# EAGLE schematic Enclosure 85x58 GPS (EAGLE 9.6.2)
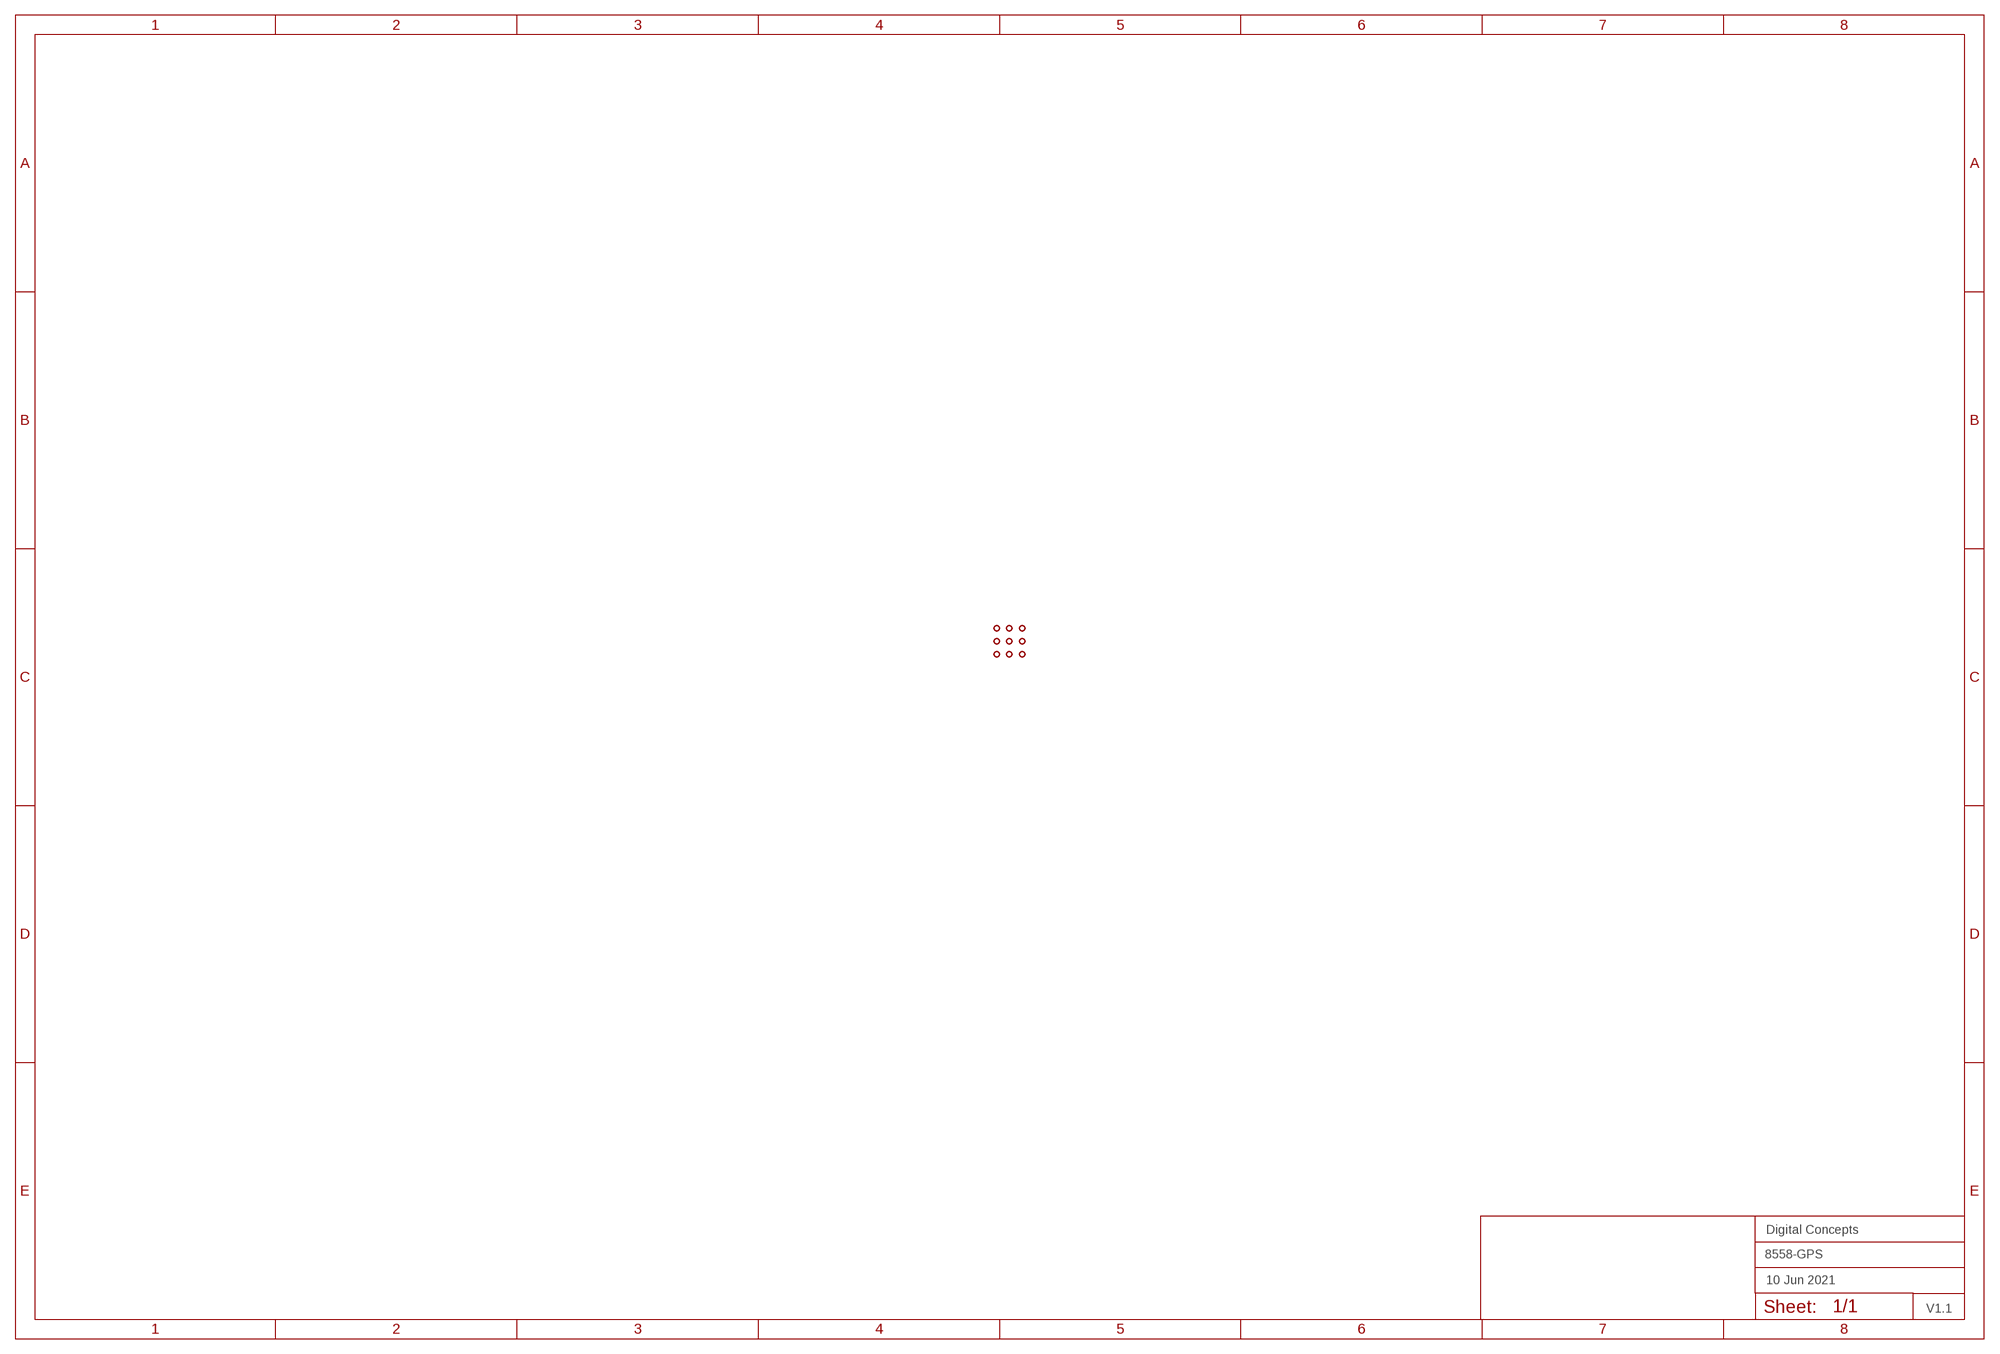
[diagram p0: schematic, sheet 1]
FRAME2 (A3L-LOC): DATE: 10 Jun 2021; OWNER: Digital Concepts; TITLE: 8558-GPS; VERSION: V1.1

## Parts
U$1  PROTO-28X18-GPS  [PROTO-28X18-GPS]

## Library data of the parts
U$1 = digitalconcepts:PROTO-28X18-GPS: 28 x 18 Prototyping board to fit an 85 x 58 enclosure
